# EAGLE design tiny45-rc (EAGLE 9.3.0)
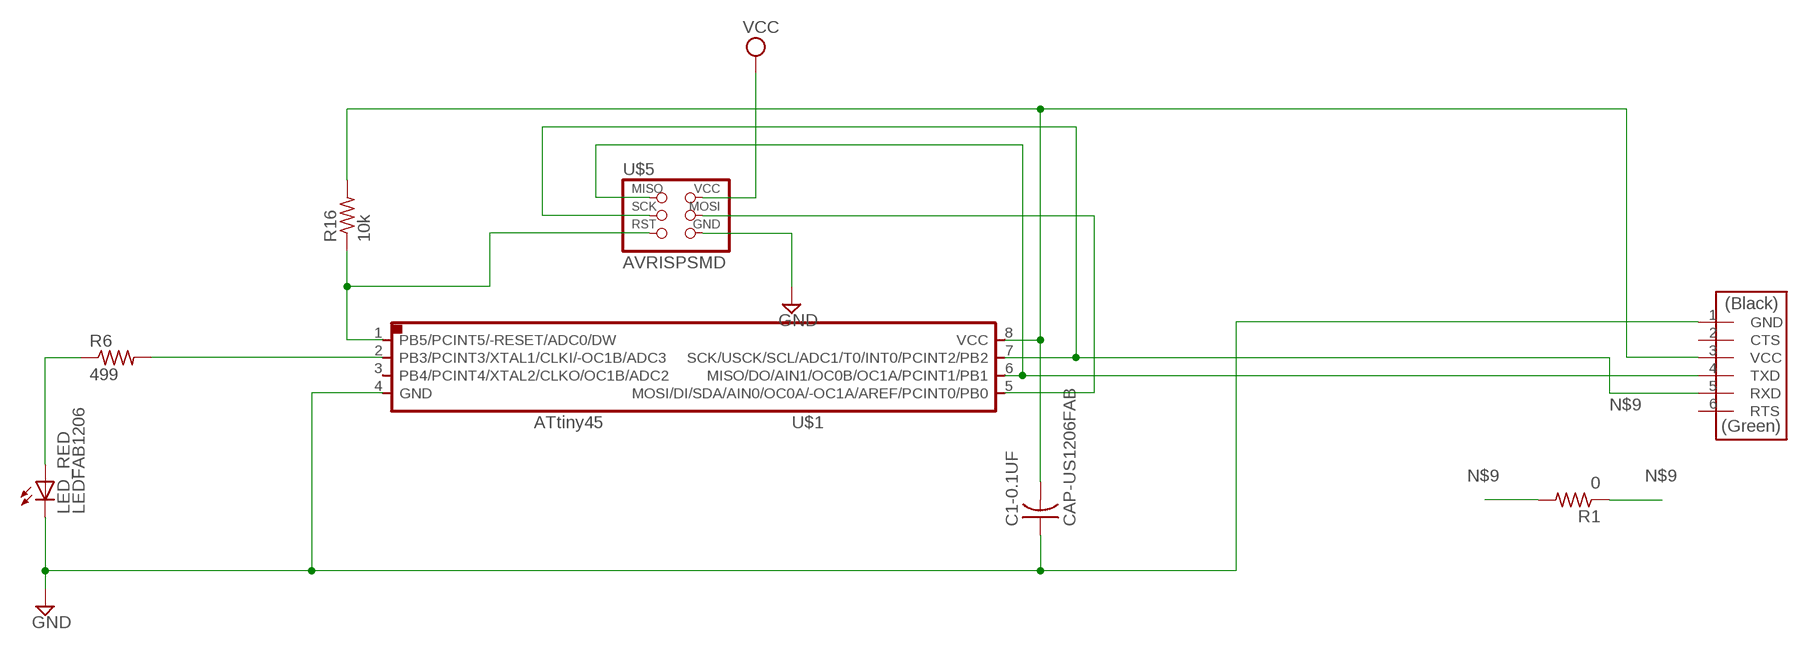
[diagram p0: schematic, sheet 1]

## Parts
C1-0.1UF  CAP-US1206FAB  [C1206FAB]
LED_RED  LEDFAB1206  [LED1206FAB]
R1  0  RES-US1206FAB  [R1206FAB]
R6  499  RES-US1206FAB  [R1206FAB]
R16  10k  RES-US1206FAB  [R1206FAB]
U$1  ATTINY45SI  [SOIC8]
U$3  FTDI-SMD-HEADER  [1X06SMD]
U$5  AVRISPSMD  [2X03SMD]

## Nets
GND: C1-0.1UF.1 LED_RED.2(C) U$1.4(GND) U$3.1(GND) U$5.6(GND)
N$1: R6.2 U$1.2(PB3/PCINT3/XTAL1/CLKI/-OC1B/ADC3)
N$2: LED_RED.1(A) R6.1
N$9: R1.1 R1.2 U$1.7(SCK/USCK/SCL/ADC1/T0/INT0/PCINT2/PB2) U$3.5(RXD) U$5.3(SCK)
N$10: U$1.6(MISO/DO/AIN1/OC0B/OC1A/PCINT1/PB1) U$3.4(TXD) U$5.1(MISO)
N$11: C1-0.1UF.2 R16.2 U$1.8(VCC) U$3.3(VCC)
N$20: R16.1 U$1.1(PB5/PCINT5/-RESET/ADC0/DW) U$5.5(RST)
N$24: U$1.5(MOSI/DI/SDA/AIN0/OC0A/-OC1A/AREF/PCINT0/PB0) U$5.4(MOSI)
VCC: U$5.2(VCC)
Unconnected: U$1.3(PB4/PCINT4/XTAL2/CLKO/OC1B/ADC2) U$3.2(CTS) U$3.6(RTS)

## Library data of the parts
C1-0.1UF = fab:CAP-US
LED_RED = fab:LED: LED
R1 R6 R16 = fab:RES-US: Resistor (US Symbol)
U$1 = fab:ATTINY45
U$3 = fab:FTDI-SMD-HEADER
U$5 = fab:AVRISP

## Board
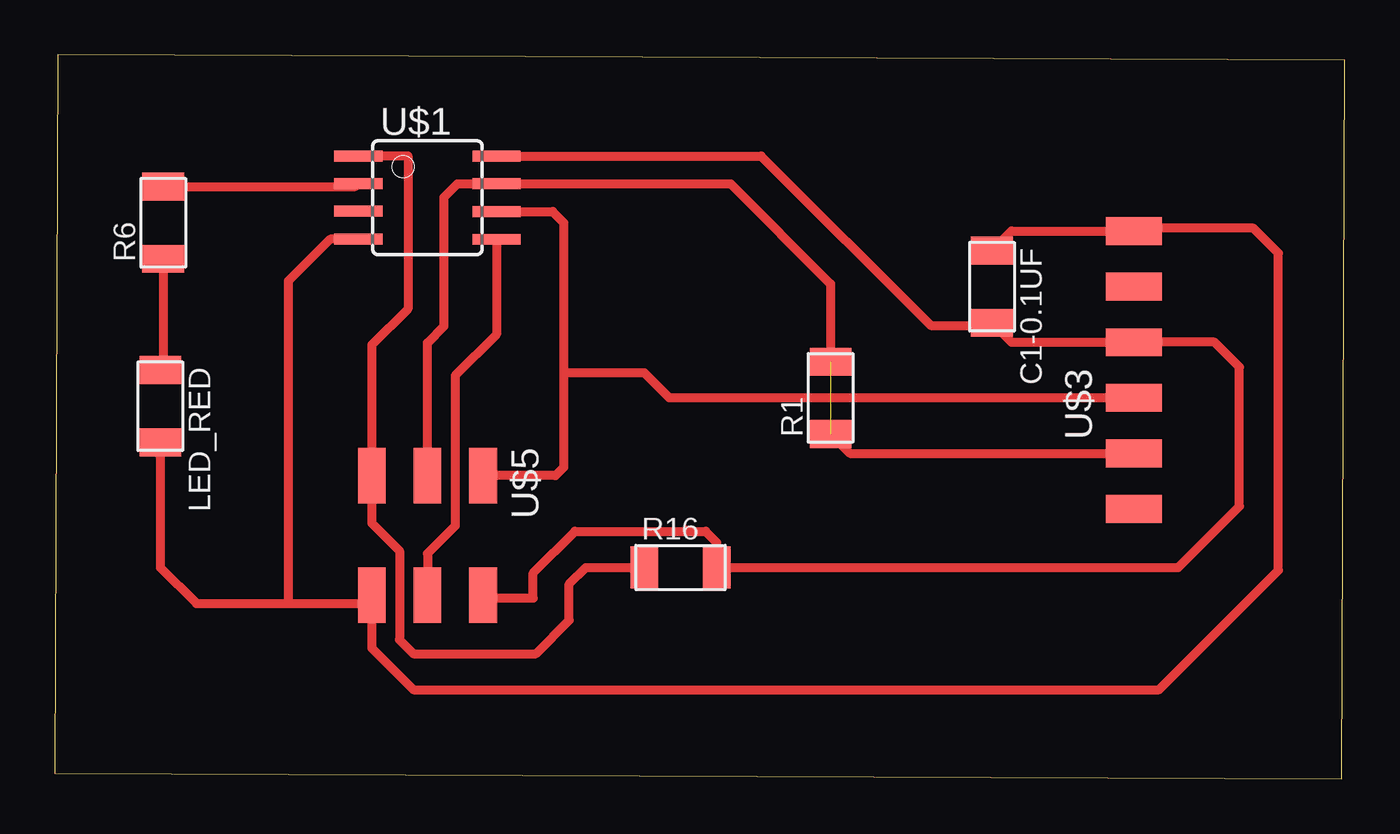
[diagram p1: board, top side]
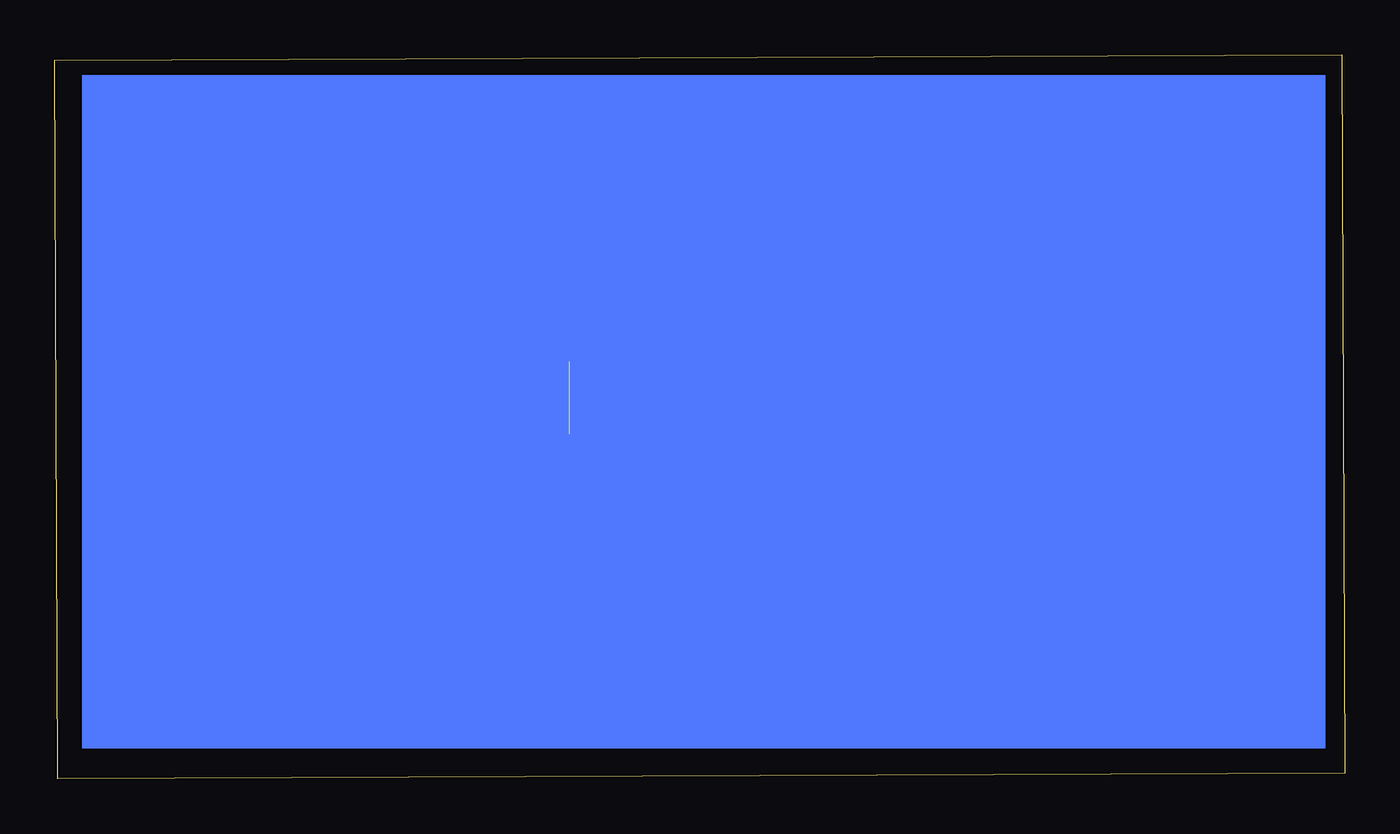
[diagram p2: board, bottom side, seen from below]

Size 58.91 x 33.07 mm. Coordinates in mm from the lower left corner, seen from the top.
Outline: 0,0.25 58.78,0 58.91,32.82 0.13,33.07 0,0.25
Copper layers (1*16): Top 0.035mm / dielectric 1.5mm / Bottom 0.035mm
Design rules "default": minimum track width 6mil, minimum drill 0.35mm, track to track 6mil, track to pad 6mil, pad to pad 6mil, via to via 6mil, smd to smd 6mil, copper to edge 40mil, drill to drill 6mil, minimum pad ring 10mil, minimum via ring 8mil, stop-mask expansion 4mil, vias tented up to drill 0mil, thermal gap 10mil

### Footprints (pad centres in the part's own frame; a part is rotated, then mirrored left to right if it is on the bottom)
C1206FAB = smd 1.27 x 1.905: 1 -1.651,0; 2 1.651,0
LED1206FAB = smd 1.27 x 1.905: 1 -1.651,0; 2 1.651,0
R1206FAB = smd 1.27 x 1.905: 1 -1.651,0; 2 1.651,0
SOIC8 = smd 0.5 x 2.2: 1 -1.905,-3.154; 2 -0.645,-3.154; 3 0.625,-3.154; 4 1.895,-3.154; 5 1.905,3.154; 6 0.635,3.154; 7 -0.635,3.154; 8 -1.905,3.154
1X06SMD = smd 2.54 x 1.27: 1 0,6.35; 2 0,3.81; 3 0,1.27; 4 0,-1.27; 5 0,-3.81; 6 0,-6.35
2X03SMD = smd 2.54 x 1.27: 1 -2.54,2.54; 2 2.92,2.54; 3 -2.54,0; 4 2.92,0; 5 -2.54,-2.54; 6 2.92,-2.54

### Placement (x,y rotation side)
C1-0.1UF  42.8,22.48 270 top
LED_RED  4.83,17.02 270 top
R1  35.43,17.4 90 top
R6  4.95,25.4 90 top
R16  28.57,9.65 0 top
U$1  17.02,26.54 270 top
U$3  49.28,18.67 0 top
U$5  17.02,11.3 270 top

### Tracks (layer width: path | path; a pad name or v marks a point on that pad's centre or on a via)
GND
  Top 0.152: 14.63,8 U$5.6 | 13.97,24.66 U$1.4
  Top 0.406: 10.67,8 6.48,8 4.83,9.65 LED_RED.2 | 10.67,8 14.63,8 | U$1.4 12.58,24.65 10.67,22.73 10.67,8 | C1-0.1UF.1 43.69,25.02 U$3.1 49.4,25.15 54.74,25.15 55.88,24 55.88,9.53 50.42,4.06 16.38,4.06 14.48,5.97 U$5.6
N$1
  Top 0.406: R6.2 13.73,27.05 U$1.2
N$2
  Top 0.406: R6.1 4.95,18.8 LED_RED.1
N$9  (1 unrouted)
  Top 0.152: U$3.5 49.23,14.86
  Top 0.406: U$5.3 17.02,19.91 17.77,20.67 17.77,26.56 18.39,27.18 U$1.7 30.86,27.18 35.43,22.61 R1.2 | 49.4,14.99 U$3.5 36.32,14.86 R1.1
N$10
  Top 0.152: 20.22,25.88 U$1.6
  Top 0.406: U$1.6 22.73,25.91 23.24,25.4 23.24,18.54 | 23.24,18.54 23.24,14.22 22.86,13.84 U$5.1 | 23.24,18.54 26.92,18.54 28.07,17.4 U$3.4
N$11
  Top 0.406: C1-0.1UF.2 42.93,20.7 | 42.93,20.7 43.69,19.94 U$3.3 52.96,19.94 54.1,18.8 54.1,12.45 51.31,9.65 R16.2 | U$1.8 32.26,28.45 40.01,20.7 42.93,20.7
N$20
  Top 0.152: 13.97,28.32 U$1.1
  Top 0.406: U$1.1 16.13,28.45 16.13,21.46 14.48,19.81 U$5.5 14.48,11.68 15.75,10.41 15.75,6.35 16.38,5.72 21.97,5.72 23.49,7.24 23.49,8.89 24.26,9.65 R16.1
N$24
  Top 0.406: U$1.5 20.17,20.3 18.29,18.41 18.29,11.56 17.02,10.29 U$5.4
VCC
  Top 0.406: U$5.2 19.69,8.26 21.84,8.26 21.84,9.4 23.75,11.3 28.83,11.3 | 28.83,11.3 29.72,11.3 30.23,10.79 | 28.83,11.3 28.88,11.35
(copper drawn outside any net)
  shapes: Bottom area x1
